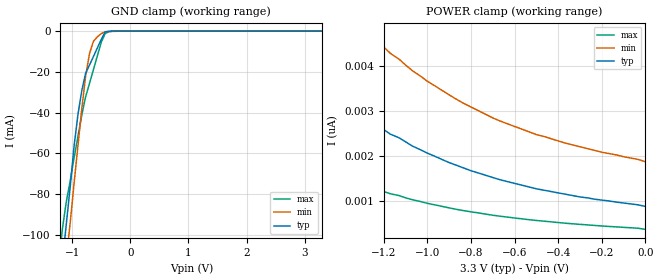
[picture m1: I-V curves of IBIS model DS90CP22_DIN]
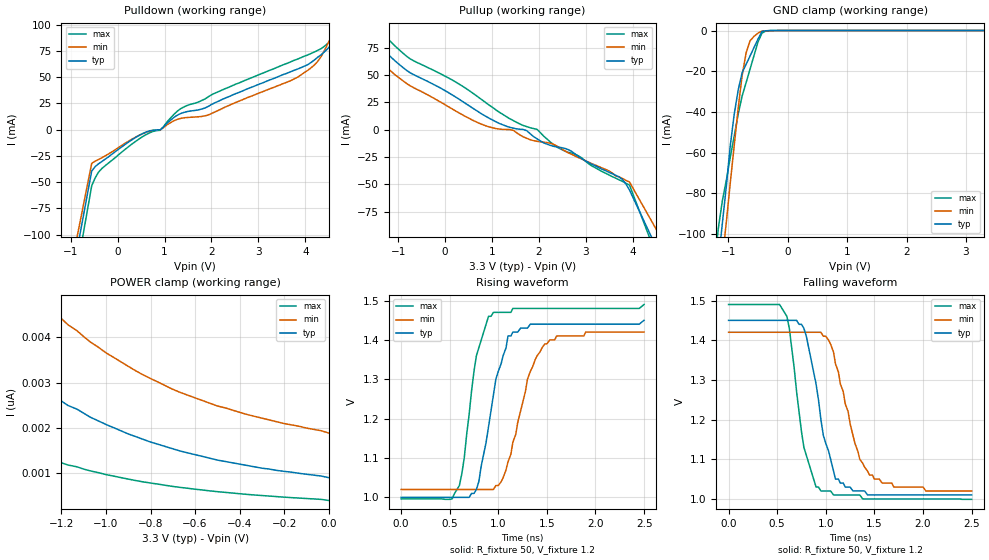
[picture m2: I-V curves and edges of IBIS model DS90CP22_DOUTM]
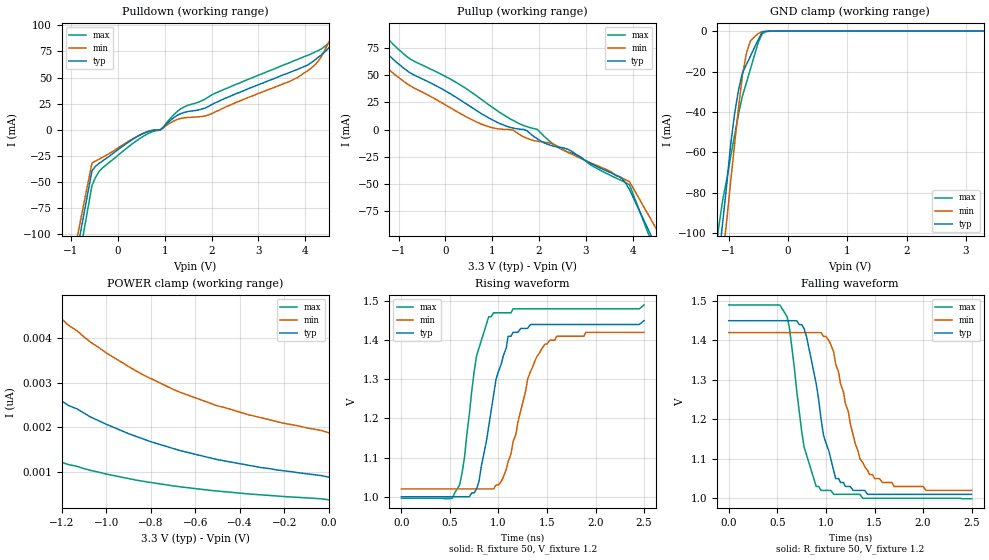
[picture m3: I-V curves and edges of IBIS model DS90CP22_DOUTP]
|   National Semiconductor Corporation
|   IBIS Model of DS90CP22M8
|   2 X 2 800 Mbps LVDS Crosspoint Switch
|   16 Lead SOIC Package
[IBIS Ver]   3.2
[Comment Char]   |_char
[File name]   ds90cp22m8.ibs
[File Rev]   2.2
[Date]   12/19/03
[Source]
SPICE to IBIS Translation
[Notes]
Created by Tim Coyle
Rev. 2.2:
- DOUT models completely re-done for the 100 ohm load (by DG)
Rev. 2.1:
- Changed Rref from 75 Ohms to 37.5 Ohms for DOUTP Model
[Disclaimer]
(C) Copyright National Semiconductor Corporation 2002
   All rights reserved
   National Semiconductor Corporation hereby grants
the user of this IBIS model a non-exclusive, nontransferable
license to use this IBIS model under the following terms.
Before using this IBIS model, the user should read this
license.  If the user does not accept these terms,  the
IBIS model should be returned to National within 30 days.
   The user is granted this license only to use the
IBIS model and is not granted rights to sell, load, rent,
lease or license the IBIS model in whole or in part, or in
modified form to anyone other than user. User may modify
the IBIS model to suit its specific applications but rights
to derivative works and such modifications shall belong to
National.
   This IBIS model is provided on an "AS IS" basis and
National makes absolutely no warranty with respect to the
information contained herein.NATIONAL DISCLAIMS AND CUSTOMER
WAIVES ALL WARRANTIES, EXPRESS OR IMPLIED, INCLUDING
WARRANTIES OF MERCHANTABILITY OR FITNESS FOR A PARTICULAR
PURPOSE. The entire risk as to quality and performance is
with the Customer. ACCORDINGLY, IN NO EVENT SHALL THE
COMPANY BE LIABLE FOR ANY DAMAGES, WHETHER IN CONTRACT OR
TORT,INCLUDING ANY LOST PROFITS OR OTHER INCIDENTAL,
CONSEQUENTIAL, EXEMPLARY, OR PUNITIVE DAMAGES ARISING OUT
OF THE USE OR APPLICATION OF THE IBIS model provided in
this package.Further, National reserves the right to make
changes without notice to any product herein to improve
reliability, function, or design. National does not convey
any license under patent rights or any other intellectual
property rights, including those of third parties.
   National is not obligated to provide maintenance or support
for the licensed IBIS model.
Contact National at ATTN:INTERFACE APPLICATIONS/IBIS MODELS.
5 Foden Road, M/S 03-03, South Porltand, ME 04106
(207) 541-6031
[Copyright]
(c) Copyright 2002 National Semiconductor Corp.
[Component]   DS90CP22M8
Si_location Pin
Timing_location Pin
[Manufacturer]   National Semiconductor Corp.
[Package]
|   TYP   MIN   MAX
R_pkg   50.0m   50.0m   50.0m
L_pkg   1.37nH   0.95n   2.07n
C_pkg   0.26pF   0.146p   0.429p
[Pin]   signal_name   model_name   R_pin   L_pin   C_pin
1   SEL1   DS90CP22_CONTROL   50.0m   2.07n   0.429p
2   SEL0   DS90CP22_CONTROL   50.0m   1.49n   0.306p
3   IN0+   DS90CP22_DIN   50.0m   0.95n   0.146p
4   IN0-   DS90CP22_DIN   50.0m   0.95n   0.152p
5   VCC   POWER   50.0m   0.95n   0.152p
6   IN1+   DS90CP22_DIN   50.0m   0.95n   0.146p
7   IN1-   DS90CP22_DIN   50.0m   1.49n   0.306p
8   NC   NC   50.0m   2.07n   0.429p
9   NC   NC   50.0m   2.07n   0.429p
10   OUT1-   DS90CP22_DOUTM   50.0m   1.49n   0.306p
11   OUT1+   DS90CP22_DOUTP   50.0m   0.95n   0.146p
12   GND   GND   50.0m   0.95n   0.152p
13   OUT0-   DS90CP22_DOUTM   50.0m   0.95n   0.152p
14   OUT0+   DS90CP22_DOUTP   50.0m   0.95n   0.146p
15   EN1   DS90CP22_CONTROL   50.0m   1.49n   0.306p
16   EN0   DS90CP22_CONTROL   50.0m   2.07n   0.429p
[Diff Pin] inv_pin vdiff   tdelay_typ tdelay_min tdelay_max
| The '+' pin is Diff_pin and the '-' pin is the inv_pin
| Vth/Vtl of Reciever = 100mv
3   4   100mv   0   0   0
6   7   100mv   0   0   0
11   10   0   0   0   0
14   13   0   0   0   0
| Models and submodels in the file (4): DS90CP22_DIN (Input), DS90CP22_DOUTM (3-state), DS90CP22_DOUTP (3-state), DS90CP22_CONTROL (Input)
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[Model]   DS90CP22_DIN
Model_type Input
Vinh=.1
Vinl=-.1
C_comp   2.49pF   2.49pF   2.49pF
[Temperature Range] 25   85   -40
[Voltage Range]   3.3   3.0   3.6
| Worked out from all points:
|   GND clamp passes 1 mA (typ) near -0.44 V on its own axis
[GND Clamp]
|V(groundclamp)   I(typ)   I(min)   I(max)
-3.3V     -803mA     -823mA     -782mA
-1.17V    -114mA     -132mA     -97.7mA
-1.1V     -94.8mA    -112mA     -83.7mA
-1.03V    -75.7mA    -93.4mA    -73.1mA
-967mV    -56.7mA    -75mA      -62.4mA
-900mV    -41.1mA    -56.5mA    -51.8mA
-833mV    -29.2mA    -38.1mA    -41.1mA
-767mV    -20.7mA    -22.1mA    -32.2mA
-700mV    -16.6mA    -11mA      -25.6mA
-633mV    -12.5mA    -5.01mA    -18.9mA
-433mV    -470uA     -263uA     -1.31mA
3.3V      923pA      1.92nA     295pA
[POWER Clamp]
|Vtable   I(typ)   I(min)   I(max)
-3.3V     38.3nA     45.4nA     26.1nA
-2.17V    9.04nA     12.9nA     4.91nA
-2.13V    8.68nA     12.5nA     4.68nA
-2.07V    7.94nA     11.6nA     4.23nA
-1.87V    6.06nA     9.14nA     3.12nA
-1.7V     4.86nA     7.56nA     2.44nA
-1.47V    3.61nA     5.85nA     1.75nA
-1.27V    2.82nA     4.74nA     1.34nA
-1V       2.07nA     3.66nA     958pA
-700mV    1.53nA     2.85nA     695pA
-500mV    1.28nA     2.48nA     579pA
0V        889pA      1.88nA     383pA
[Model]   DS90CP22_DOUTM
Model_type 3-state
Enable Active-High
Polarity Inverting
Vref=1.2
Vmeas=1.2
Rref=50   | 100 Ohms Across Outputs OUTP and OUTM
Cref=5p
C_comp   3.493pF   3.493pF   3.493pF
[Temperature Range] 25   85   -40
[Voltage Range]   3.3   3.0   3.6
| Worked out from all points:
|   slope of the pulldown table from 0 to 0.495 V, typ, clamps not added: 33.8 ohm
|   slope of the pullup table from 0 to 0.495 V, typ, clamps not added: 37.2 ohm
|   GND clamp passes 1 mA (typ) near -0.44 V on its own axis
|   falling waveform, R_fixture 50, V_fixture 1.2: 20-80 % time 212ps typ, 250ps min, 172ps max; typ from 1.45 V to 1.01 V
|   rising waveform, R_fixture 50, V_fixture 1.2: 20-80 % time 217ps typ, 250ps min, 167ps max; typ from 1 V to 1.45 V
[Pullup]
|Vtable   I(typ)   I(min)   I(max)
-3.3V     282mA      249mA      331mA
-1.69V    113mA      101mA      125mA
-1.62V    104mA      93.1mA     115mA
-1.48V    87.5mA     77.5mA     98.1mA
-1.26V    70.3mA     58.2mA     84.4mA
-1.04V    61.8mA     49.2mA     75.3mA
569mV     20.2mA     9.05mA     34mA
1.96V     -8.33mA    -10.6mA    315uA
2.32V     -15.2mA    -13.5mA    -13.9mA
3.56V     -40.2mA    -39.4mA    -42.8mA
3.93V     -55.1mA    -47.8mA    -50.6mA
6.6V      -300mA     -250mA     -350mA
[Pulldown]
|V(pulldown)   I(typ)   I(min)   I(max)
-3.3V     -700mA     -650mA     -750mA
-554mV    -39.4mA    -32mA      -53.4mA
-335mV    -30.2mA    -26.6mA    -36.8mA
468mV     -5.17mA    -5.08mA    -8.42mA
906mV     -142uA     -92.7uA    -509uA
1.34V     15.4mA     10.8mA     20mA
1.93V     22.2mA     14.1mA     31.3mA
3.83V     57.7mA     49.9mA     67.2mA
4.26V     68.9mA     64.9mA     75.5mA
4.7V      94.1mA     103mA      91.8mA
4.85V     110mA      116mA      100mA
6.6V      249mA      159mA      346mA
[GND Clamp]
-3.3V     -803mA     -823mA     -782mA
-1.17V    -114mA     -132mA     -97.7mA
-1.1V     -94.8mA    -112mA     -83.7mA
-1.03V    -75.7mA    -93.4mA    -73.1mA
-967mV    -56.7mA    -75mA      -62.4mA
-900mV    -41.1mA    -56.5mA    -51.8mA
-833mV    -29.2mA    -38.1mA    -41.1mA
-767mV    -20.7mA    -22.1mA    -32.2mA
-700mV    -16.6mA    -11mA      -25.6mA
-633mV    -12.5mA    -5.01mA    -18.9mA
-433mV    -470uA     -263uA     -1.31mA
3.3V      923pA      1.92nA     295pA
[POWER Clamp]
-3.3V     38.3nA     45.4nA     26.1nA
-2.17V    9.04nA     12.9nA     4.91nA
-2.13V    8.68nA     12.5nA     4.68nA
-2.07V    7.94nA     11.6nA     4.23nA
-1.87V    6.06nA     9.14nA     3.12nA
-1.7V     4.86nA     7.56nA     2.44nA
-1.47V    3.61nA     5.85nA     1.75nA
-1.27V    2.82nA     4.74nA     1.34nA
-1V       2.07nA     3.66nA     958pA
-700mV    1.53nA     2.85nA     695pA
-500mV    1.28nA     2.48nA     579pA
0V        889pA      1.88nA     383pA
[Ramp]
dV/dt_r   240mV/.292ns   200mV/.430ns   280mV/.220ns
dV/dt_f   240mv/.300ns   200mv/.400ns   280mv/.220ns
R_load=50
[Falling Waveform]
R_fixture=50
V_fixture=1.2
V_fixture_min=1.2
V_fixture_max=1.2
| Time   V(typ)  V(min)  V(max)
0s        1.45V      1.42V      1.49V
525ps     1.45V      1.42V      1.49V
600ps     1.45V      1.42V      1.46V
775ps     1.43V      1.42V      1.13V
900ps     1.29V      1.42V      1.03V
950ps     1.2V       1.42V      1.02V
1.1ns     1.05V      1.34V      1.01V
1.3ns     1.02V      1.14V      1.01V
1.45ns    1.01V      1.06V      1V
2.5ns     1.01V      1.02V      999mV
[Rising Waveform]
R_fixture=50
V_fixture=1.2
V_fixture_min=1.2
V_fixture_max=1.2
| Time   V(typ)  V(min)  V(max)
0s        1V         1.02V      996mV
525ps     1V         1.02V      996mV
600ps     1V         1.02V      1.03V
650ps     1V         1.02V      1.1V
775ps     1.02V      1.02V      1.36V
950ps     1.26V      1.02V      1.47V
1.1ns     1.41V      1.09V      1.47V
1.3ns     1.43V      1.3V       1.48V
1.48ns    1.44V      1.39V      1.48V
2.5ns     1.45V      1.42V      1.49V
[Model]   DS90CP22_DOUTP
Model_type 3-state
Enable Active-High
Polarity Non-Inverting
Vref=1.2
Vmeas=1.2
Rref=50   | 100 ohms across outputs OUTP and OUTM
Cref=5p
C_comp   3.493pF   3.493pF   3.493pF
[Temperature Range] 25   85   -40
[Voltage Range]   3.3   3.0   3.6
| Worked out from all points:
|   slope of the pulldown table from 0 to 0.495 V, typ, clamps not added: 33.8 ohm
|   slope of the pullup table from 0 to 0.495 V, typ, clamps not added: 37.2 ohm
|   GND clamp passes 1 mA (typ) near -0.44 V on its own axis
|   falling waveform, R_fixture 50, V_fixture 1.2: 20-80 % time 212ps typ, 250ps min, 172ps max; typ from 1.45 V to 1.01 V
|   rising waveform, R_fixture 50, V_fixture 1.2: 20-80 % time 217ps typ, 250ps min, 167ps max; typ from 1 V to 1.45 V
[Pullup]
|Vtable   I(typ)   I(min)   I(max)
-3.3V     282mA      249mA      331mA
-1.69V    113mA      101mA      125mA
-1.62V    104mA      93.1mA     115mA
-1.48V    87.5mA     77.5mA     98.1mA
-1.26V    70.3mA     58.2mA     84.4mA
-1.04V    61.8mA     49.2mA     75.3mA
569mV     20.2mA     9.05mA     34mA
1.96V     -8.33mA    -10.6mA    315uA
2.32V     -15.2mA    -13.5mA    -13.9mA
3.56V     -40.2mA    -39.4mA    -42.8mA
3.93V     -55.1mA    -47.8mA    -50.6mA
6.6V      -300mA     -250mA     -350mA
[Pulldown]
|V(pulldown)   I(typ)   I(min)   I(max)
-3.3V     -700mA     -650mA     -750mA
-554mV    -39.4mA    -32mA      -53.4mA
-335mV    -30.2mA    -26.6mA    -36.8mA
468mV     -5.17mA    -5.08mA    -8.42mA
906mV     -142uA     -92.7uA    -509uA
1.34V     15.4mA     10.8mA     20mA
1.93V     22.2mA     14.1mA     31.3mA
3.83V     57.7mA     49.9mA     67.2mA
4.26V     68.9mA     64.9mA     75.5mA
4.7V      94.1mA     103mA      91.8mA
4.85V     110mA      116mA      100mA
6.6V      249mA      159mA      346mA
[GND Clamp]
-3.3V     -803mA     -823mA     -782mA
-1.17V    -114mA     -132mA     -97.7mA
-1.1V     -94.8mA    -112mA     -83.7mA
-1.03V    -75.7mA    -93.4mA    -73.1mA
-967mV    -56.7mA    -75mA      -62.4mA
-900mV    -41.1mA    -56.5mA    -51.8mA
-833mV    -29.2mA    -38.1mA    -41.1mA
-767mV    -20.7mA    -22.1mA    -32.2mA
-700mV    -16.6mA    -11mA      -25.6mA
-633mV    -12.5mA    -5.01mA    -18.9mA
-433mV    -470uA     -263uA     -1.31mA
3.3V      923pA      1.92nA     295pA
[POWER Clamp]
-3.3V     38.3nA     45.4nA     26.1nA
-2.17V    9.04nA     12.9nA     4.91nA
-2.13V    8.68nA     12.5nA     4.68nA
-2.07V    7.94nA     11.6nA     4.23nA
-1.87V    6.06nA     9.14nA     3.12nA
-1.7V     4.86nA     7.56nA     2.44nA
-1.47V    3.61nA     5.85nA     1.75nA
-1.27V    2.82nA     4.74nA     1.34nA
-1V       2.07nA     3.66nA     958pA
-700mV    1.53nA     2.85nA     695pA
-500mV    1.28nA     2.48nA     579pA
0V        889pA      1.88nA     383pA
[Ramp]
dV/dt_r   240mV/.292ns   200mV/.430ns   280mV/.220ns
dV/dt_f   240mv/.300ns   200mv/.400ns   280mv/.220ns
R_load=50
[Falling Waveform]
R_fixture=50
V_fixture=1.2
V_fixture_min=1.2
V_fixture_max=1.2
| Time   V(typ)  V(min)  V(max)
0s        1.45V      1.42V      1.49V
525ps     1.45V      1.42V      1.49V
600ps     1.45V      1.42V      1.46V
775ps     1.43V      1.42V      1.13V
900ps     1.29V      1.42V      1.03V
950ps     1.2V       1.42V      1.02V
1.1ns     1.05V      1.34V      1.01V
1.3ns     1.02V      1.14V      1.01V
1.45ns    1.01V      1.06V      1V
2.5ns     1.01V      1.02V      999mV
[Rising Waveform]
R_fixture=50
V_fixture=1.2
V_fixture_min=1.2
V_fixture_max=1.2
| Time   V(typ)  V(min)  V(max)
0s        1V         1.02V      996mV
525ps     1V         1.02V      996mV
600ps     1V         1.02V      1.03V
650ps     1V         1.02V      1.1V
775ps     1.02V      1.02V      1.36V
950ps     1.26V      1.02V      1.47V
1.1ns     1.41V      1.09V      1.47V
1.3ns     1.43V      1.3V       1.48V
1.48ns    1.44V      1.39V      1.48V
2.5ns     1.45V      1.42V      1.49V
